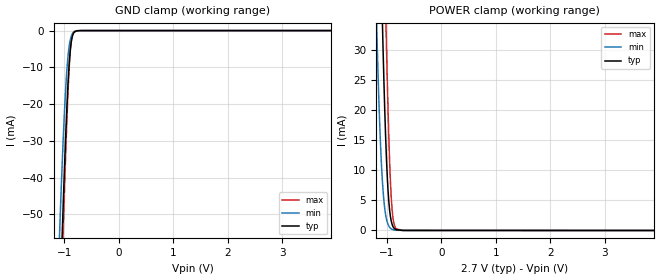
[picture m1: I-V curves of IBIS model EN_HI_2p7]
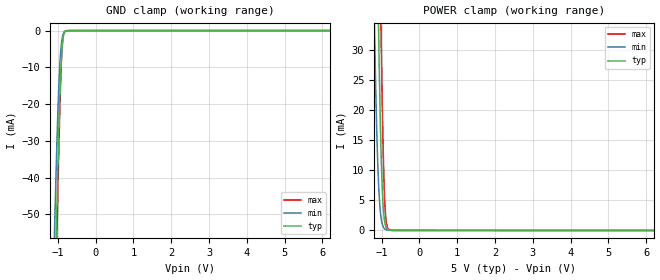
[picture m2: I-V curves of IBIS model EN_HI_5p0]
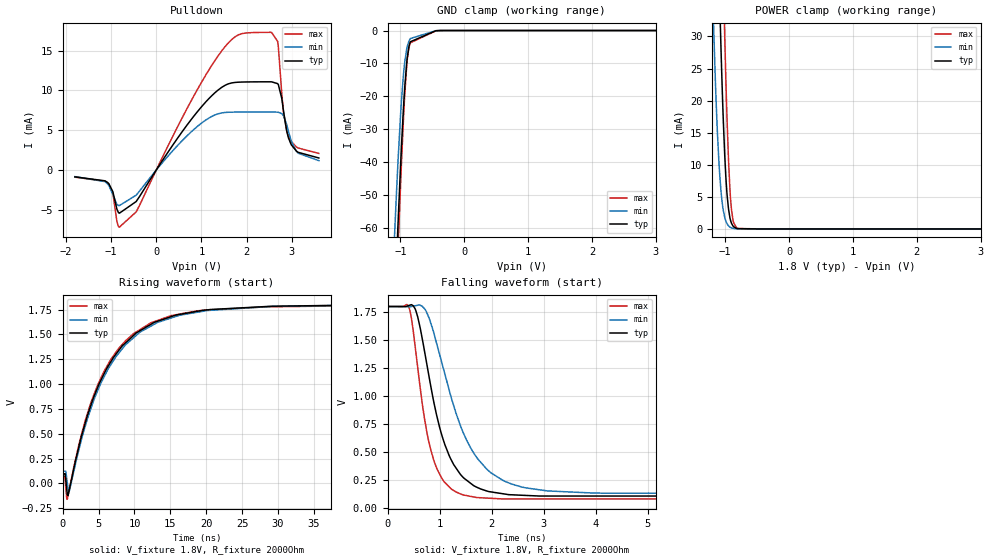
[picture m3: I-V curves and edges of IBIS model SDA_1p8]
|Texas Instruments Incorporated
| Marketing part#   Digital Voltage Range   Package-type   #pins
|   TUSB320H   2.7V - 5.0V   X2QFN   12
[IBIS Ver]   4.1
[File name]   tusb320h.ibs
[File Rev]   1.0
[Date]   08/17/2015
[Source]
| Texas Instruments Incorporated.
| 12500 TI Blvd
| Dallas, TX -75243
[Notes]   Revision History:
| Rev 1.0: 08/17/2015
| - Initial version of the model
| - Model generated from simulations in TISPICE
| - C_comp although listed in numerical order of value are
|   obtained from varying PVT conditions. For PVT conditions for
|   each specific value refer the buffer description under
|   respective [Model]. IBIS model user is responsible for using
|   appropriate C_comp to simulate for Signal Integrity.
| - Warnings regarding combined Non-monotonicity of various models have been
|   reviewd and considered minor and can be ignored.
| - Model names with a trailing _2p7 contain the model for
|   2.7V operation. Model names with a trailing _5p0 contain the model
|   for 5.0V operation.
| - CC1 and CC2 pin have a number of models depending pull-up and pull-down
|   cases (pu_xxx_xxx and pd_xxx respectively). Pull-up model also features
|   dependng on the strength of pull up (pu_xxx_80u, pu_xxx_180u and
|   pu_xxx_330u).
[Disclaimer]
| This model is designed as an aid for customers of Texas Instruments.
| TI and its licensors and suppliers make no warranties, either expressed
| or implied, with respect to this  model, including the warranties of
| merchantability or fitness for a particular purpose. The model is
| provided solely on an "as is" basis. The entire risk as to its quality
| and performance is with the customer.
[Copyright]
 (C) Copyright 2015 Texas Instruments Incorporated.All rights reserved.
|   Device
[Component]  TUSB320H
[Manufacturer]   TI
[Package]  |X2QFN   12
|   typ   min   max
R_pkg   0.067   0.027   0.083
L_pkg   0.937nH   0.593nH   1.143nH
C_pkg   0.144pF   0.126pF   0.200pF
[Pin]  signal_name   model_name   R_pin   L_pin   C_pin
1   CC1   CC   NA   NA   NA
2   CC2   CC   NA   NA   NA
3   PORT   ADDR   NA   NA   NA
4   VBUS_DET   NC   NA   NA   NA
5   ADDR   ADDR   NA   NA   NA
6   INT_N/OUT3   INT   NA   NA   NA
7   SDA/OUT1   SDA   NA   NA   NA
8   SCL/OUT2   SDA   NA   NA   NA
9   ID   INT   NA   NA   NA
10   GND   GND   NA   NA   NA
11   EN   EN_PD   NA   NA   NA
12   VDD   POWER   NA   NA   NA
|   Model Selectors
[Model Selector]  ADDR
ADDR_5p0  ADDR input buffer at 5.0V operation.
ADDR_2p7  ADDR input buffer at 2.7V operation.
[Model Selector]  INT
INT_5p0  INT buffer at 5.0V operation.
INT_2p7  INT buffer at 2.7V operation.
[Model Selector]  SDA
SDA_3p3  SDA buffer at 3.3V operation.
SDA_1p8  SDA buffer at 1.8V operation.
[Model Selector]  CC
PD_5p0  CC1/CC2 buffer at pull-down state at 5.0V VCC.
PD_2p7  CC1/CC2 buffer at pull-down state at 2.7V VCC.
PU_5p0_80u  CC1/CC2 buffer at 80uA pull-up state at 5.0V VCC.
PU_5p0_180u  CC1/CC2 buffer at 180uA pull-up state at 5.0V VCC.
PU_5p0_330u  CC1/CC2 buffer at 330uA pull-up state at 5.0V VCC.
PU_2p7_80u  CC1/CC2 buffer at 80uA pull-up state at 2.7V VCC.
PU_2p7_180u  CC1/CC2 buffer at 180uA pull-up state at 2.7V VCC.
PU_3p5_330u  CC1/CC2 buffer at 330uA pull-up state at 3.5V VCC.
[Model Selector]  EN_PD
EN_HI_5p0  EN input buffer at 5.0V operation.
EN_HI_2p7  EN input buffer at 2.7V operation.
| Models and submodels in the file (16): EN_HI_2p7 (Input), EN_HI_5p0 (Input), SDA_1p8 (I/O_open_drain), SDA_3p3 (I/O_open_drain), PU_3p5_330u (Input), PU_5p0_330u (Input), PU_5p0_180u (Input), PU_5p0_80u (Input), PU_2p7_180u (Input), PU_2p7_80u (Input), PD_5p0 (Input), PD_2p7 (Input), INT_5p0 (Open_drain), INT_2p7 (Open_drain), ADDR_5p0 (Input), ADDR_2p7 (Input)
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|   Model
[Model]   EN_HI_2p7
Model_type   Input
Vinl = 0.81
Vinh = 1.89
|   typ   min   max
C_comp   0.453pF   0.4pF   0.56pF
[Voltage Range]   2.7   2.699   2.701
[Temperature Range]   27   105   -40
[Power Clamp Reference]   2.7   2.699   2.701
[GND Clamp Reference]   0   0   0
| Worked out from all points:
|   GND clamp passes 1 mA (typ) near -0.84 V on its own axis
|   POWER clamp passes 1 mA (typ) near -0.90 V on its own axis
[GND Clamp]
|   Voltage   I(typ)   I(min)   I(max)
-5V       -2.267A    -2.153A    -2.357A
-1.1V     -83.39mA   -59.91mA   -94.16mA
-1.085V   -76.15mA   -53.61mA   -86.34mA
-1.04V    -55.17mA   -35.94mA   -63.45mA
-1.025V   -48.5mA    -30.57mA   -56.07mA
-965mV    -24.37mA   -12.92mA   -28.65mA
-935mV    -14.69mA   -7.111mA   -17.09mA
-905mV    -7.498mA   -3.47mA    -8.161mA
-890mV    -4.98mA    -2.334mA   -5.039mA
-860mV    -1.923mA   -1.003mA   -1.527mA
-815mV    -376.9uA   -263.9uA   -184.7uA
10V       0A         0A         0A
[POWER Clamp]
|   Voltage   I(typ)   I(min)   I(max)
-5V       2.317A     2.221A     2.385A
-1.19V    81.56mA    34.73mA    119mA
-1.13V    53.92mA    17.15mA    87.53mA
-1.085V   35.47mA    8.498mA    65.05mA
-1.025V   15.94mA    2.685mA    37.58mA
-1.01V    12.3mA     1.959mA    31.41mA
-980mV    6.746mA    1.024mA    20.31mA
-935mV    2.282mA    377.8uA    8.072mA
-905mV    1.023mA    194.2uA    3.506mA
-875mV    446.2uA    100.9uA    1.32mA
-710mV    10.49uA    7.778uA    11.97uA
10V       0A         0A         0A
|   Model
[Model]   EN_HI_5p0
Model_type   Input
Vinl = 1.5
Vinh = 3.5
|   typ   min   max
C_comp   0.453pF   0.4pF   0.56pF
[Voltage Range]   5   4.999   5.001
[Temperature Range]   27   105   -40
[Power Clamp Reference]   5   4.999   5.001
[GND Clamp Reference]   0   0   0
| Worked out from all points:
|   GND clamp passes 1 mA (typ) near -0.84 V on its own axis
|   POWER clamp passes 1 mA (typ) near -0.90 V on its own axis
[GND Clamp]
|   Voltage   I(typ)   I(min)   I(max)
-5V       -2.267A    -2.153A    -2.357A
-1.1V     -83.39mA   -59.91mA   -94.16mA
-1.085V   -76.15mA   -53.61mA   -86.34mA
-1.04V    -55.17mA   -35.94mA   -63.45mA
-1.025V   -48.5mA    -30.57mA   -56.07mA
-965mV    -24.37mA   -12.92mA   -28.65mA
-935mV    -14.69mA   -7.111mA   -17.09mA
-905mV    -7.498mA   -3.47mA    -8.161mA
-890mV    -4.98mA    -2.334mA   -5.039mA
-860mV    -1.923mA   -1.003mA   -1.527mA
-815mV    -376.9uA   -263.9uA   -184.7uA
10V       0A         0A         0A
[POWER Clamp]
|   Voltage   I(typ)   I(min)   I(max)
-5V       2.317A     2.221A     2.385A
-1.19V    81.56mA    34.73mA    119mA
-1.13V    53.93mA    17.15mA    87.53mA
-1.085V   35.48mA    8.501mA    65.05mA
-1.025V   15.94mA    2.688mA    37.58mA
-1.01V    12.3mA     1.962mA    31.41mA
-980mV    6.75mA     1.027mA    20.31mA
-935mV    2.286mA    381.6uA    8.077mA
-905mV    1.027mA    198uA      3.511mA
-875mV    450.6uA    104.7uA    1.326mA
-710mV    15.05uA    11.62uA    18.01uA
10V       0A         0A         0A
|   Model
[Model]   SDA_1p8
Model_type   I/O_open_drain
Polarity   Non-Inverting
Enable   Active-Low
Vinl = 0.54
Vinh = 1.26
Vmeas = 0.9
Vref = 1.8
Cref = 1pF
Rref = 2000
|   typ   min   max
C_comp   1pF   1pF   1pF
[Voltage Range]   1.8   1.799   1.801
[Temperature Range]   27   105   -40
[Pullup Reference]   1.8   1.799   1.801
[Pulldown Reference]   -0   -0   0
[Power Clamp Reference]   1.8   1.799   1.801
[GND Clamp Reference]   0   0   0
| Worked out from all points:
|   slope of the pulldown table from 0 to 0.27 V, typ, clamps not added: 116 ohm
|   POWER clamp passes 1 mA (typ) near -0.90 V on its own axis
|   falling waveform, V_fixture 1.8V, R_fixture 2000Ohm: 20-80 % time 524ps typ, 753ps min, 365ps max; typ from 1.8 V to 0.097 V
|   rising waveform, V_fixture 1.8V, R_fixture 2000Ohm: 20-80 % time 6.95ns typ, 7.17ns min, 6.72ns max; typ from 0.097 V to 1.8 V
[Pulldown]
|   Voltage   I(typ)   I(min)   I(max)
-1.8V     -861.7uA   -829.5uA   -898.8uA
-1.055V   -1.697mA   -1.903mA   -1.756mA
-817.2mV  -5.43mA    -4.472mA   -7.18mA
-444.6mV  -3.959mA   -3.16mA    -5.26mA
997.2mV   7.919mA    5.873mA    10.98mA
1.575V    10.78mA    7.255mA    15.85mA
1.975V    11.07mA    7.293mA    17.21mA
2.687V    10.86mA    7.273mA    16.18mA
2.817V    7.429mA    6.821mA    7.291mA
2.925V    4.079mA    4.907mA    4.283mA
3.141V    2.229mA    2.119mA    2.769mA
3.6V      1.513mA    1.177mA    2.086mA
[GND Clamp]
|   Voltage   I(typ)   I(min)   I(max)
-1.8V     -477.7mA   -433.3mA   -503.9mA
-1.098V   -88.8mA    -65.47mA   -98.86mA
-1.06V    -70.18mA   -49.29mA   -78.84mA
-1.044V   -62.47mA   -42.77mA   -70.47mA
-1.039V   -59.94mA   -40.67mA   -67.71mA
-1.033V   -57.43mA   -38.6mA    -64.97mA
-984.6mV  -36.2mA    -22.04mA   -41.43mA
-930.6mV  -17.09mA   -9.495mA   -19.33mA
-892.8mV  -8.393mA   -4.912mA   -8.993mA
-844.2mV  -3.427mA   -2.45mA    -3.746mA
-396mV    -22.95uA   -18.2uA    -31.49uA
3.6V      0A         0A         0A
[POWER Clamp]
|   Voltage   I(typ)   I(min)   I(max)
-1.8V     416.5mA    342.1mA    467mA
-1.184V   78.87mA    32.83mA    116mA
-1.125V   51.76mA    15.98mA    84.97mA
-1.082V   34.26mA    8.033mA    63.5mA
-1.066V   28.4mA     5.989mA    55.78mA
-1.033V   18.16mA    3.173mA    41.1mA
-1.006V   11.46mA    1.801mA    29.9mA
-968.4mV  5.192mA    787uA      16.58mA
-919.8mV  1.521mA    263.6uA    5.398mA
-871.2mV  394.5uA    87.13uA    1.15mA
-795.6mV  45.22uA    15.45uA    73.94uA
3.6V      0A         0A         0A
[Ramp]
R_load = 2000
|   typ   min   max
dV/dt_r   1.0217/6.85247e-09   1.00587/7.07089e-09   1.03669/6.69844e-09
dV/dt_f   1.0217/5.23594e-10   1.00587/7.49816e-10   1.03669/3.63608e-10
[Falling Waveform]
V_fixture = 1.8V
V_fixture_min = 1.799V
V_fixture_max = 1.801V
R_fixture = 2000Ohm
C_fixture = 0F
|   Time   V(typ)   V(min)   V(max)
0s        1.8V       1.799V     1.801V
416.9ps   1.81V      1.799V     1.784V
544.7ps   1.761V     1.808V     1.386V
755.7ps   1.281V     1.743V     673.4mV
1.038ns   655.1mV    1.305V     264.8mV
1.272ns   383.6mV    910.5mV    151.4mV
1.531ns   240.2mV    592.2mV    105.5mV
2.202ns   124.2mV    247.3mV    76.92mV
4.106ns   102.7mV    128.6mV    76.88mV
200ns     97.17mV    122.5mV    73.18mV
[Rising Waveform]
V_fixture = 1.8V
V_fixture_min = 1.799V
V_fixture_max = 1.801V
R_fixture = 2000Ohm
C_fixture = 0F
|   Time   V(typ)   V(min)   V(max)
0s        97.17mV    122.5mV    73.18mV
282ps     96.16mV    122mV      72.25mV
579ps     -75.06mV   32.04mV    -161mV
903.1ps   -66.45mV   -77.41mV   -62.75mV
2.342ns   398.2mV    365.7mV    418.3mV
3.979ns   799.8mV    764.9mV    823.7mV
7.798ns   1.337V     1.31V      1.359V
13.22ns   1.632V     1.621V     1.641V
18.71ns   1.732V     1.722V     1.736V
200ns     1.8V       1.799V     1.801V
